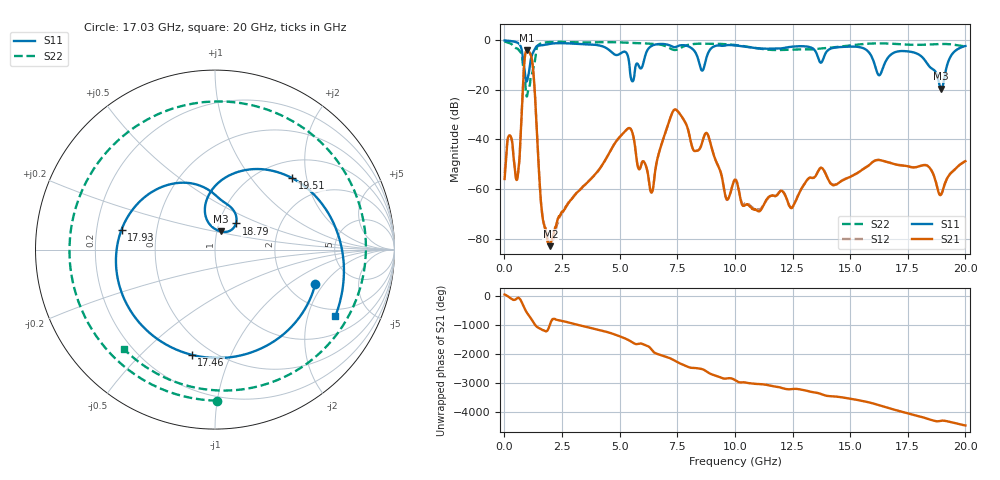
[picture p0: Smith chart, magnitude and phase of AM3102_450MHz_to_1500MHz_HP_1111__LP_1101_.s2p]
!Agilent Technologies,E8364B,MY43040894,A.07.50.67
!Agilent E8364B: A.07.50.67
!Date: Thursday, January 11, 2018 06:52:09
!Correction: S11(Full 2 Port(1,2))
!S21(Full 2 Port(1,2))
!S12(Full 2 Port(1,2))
!S22(Full 2 Port(1,2))
!S2P File: Measurements: S11, S21, S12, S22:
# Hz S  dB  R 50
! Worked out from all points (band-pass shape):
!   1601 points, 10 MHz to 20 GHz, reference 50 ohm
!   highest |S21| = -3.96 dB at 984.5 MHz (marker M1); lowest = -83.0 dB at 1.997 GHz (marker M2)
!   |S21| within 3 dB of the highest: 885 MHz to 1.176 GHz (291 MHz wide, 28.2 % of centre)
!   lowest |S11| = -19.5 dB at 18.95 GHz (marker M3), VSWR 1.24, Z = 52.1 + j10.7 ohm
!   |S11| at or under -10 dB: 5.425 GHz to 5.703 GHz (278.5 MHz wide, 5.01 % of centre); 16.07 GHz to 16.47 GHz (397 MHz wide, 2.44 % of centre); 18.39 GHz to 19.21 GHz (818.5 MHz wide, 4.35 % of centre)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
!   |S22| runs from -22.7 to -0.5 dB; largest |S21 - S12| = 0.0024
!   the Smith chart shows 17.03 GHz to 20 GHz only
!   S11 on the Smith chart (normalised r, x): 17.03 GHz: 2.82, -1.65; 17.46 GHz: 0.39, -0.72; 17.93 GHz: 0.31, +0.10; 18.79 GHz: 1.20, +0.36; 19.51 GHz: 1.36, +1.65; 20 GHz: 1.68, -3.02
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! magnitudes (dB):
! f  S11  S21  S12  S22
! 10 MHz  -0.1  -55.9  -53.5  -0.5
! 234.9 MHz  -0.3  -38.4  -38.4  -1.2
! 572.2 MHz  -1.0  -55.4  -55.3  -3.4
! 984.5 MHz  -16.4  -4.0  -4.0  -22.6
! 1.247 GHz  -4.9  -11.7  -11.7  -11.7
! 1.647 GHz  -2.0  -70.5  -70.3  -1.1
! 1.997 GHz  -1.4  -83.0  -81.6  -0.7
! 3.346 GHz  -1.5  -59.7  -59.8  -0.9
! 5.357 GHz  -6.3  -35.6  -35.6  -1.0
! 6.369 GHz  -2.4  -61.4  -61.1  -1.4
! 6.682 GHz  -1.5  -46.2  -46.2  -1.6
! 7.444 GHz  -2.7  -28.0  -28.0  -3.9
! 10.01 GHz  -2.1  -56.3  -56.1  -1.9
! 13.34 GHz  -3.1  -55.4  -55.5  -3.7
! 16.68 GHz  -6.6  -49.3  -49.2  -1.3
! 17.03 GHz  -4.6  -50.2  -50.2  -1.5
! 17.46 GHz  -4.4  -50.7  -50.7  -1.7
! 17.93 GHz  -5.5  -51.0  -51.0  -1.8
! 18.79 GHz  -14.6  -59.8  -59.6  -1.5
! 18.95 GHz  -19.5  -62.1  -62.2  -1.5
! 19.51 GHz  -4.6  -52.4  -52.3  -1.8
! 20 GHz  -2.3  -48.8  -48.7  -2.5
